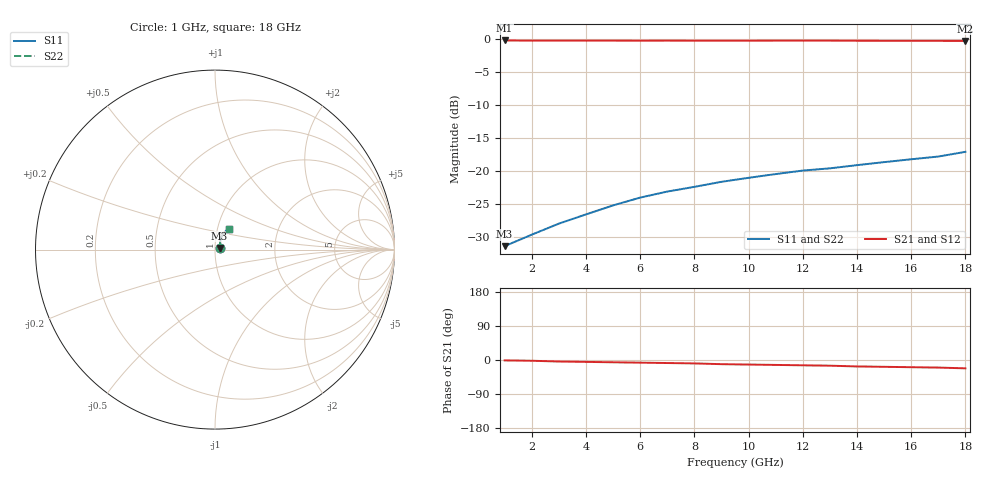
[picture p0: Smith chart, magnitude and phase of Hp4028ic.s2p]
!HPND-4028 beam lead PIN diode
!Series configuration S-parameters If=10 mA.  Last updated 10/3/97
# mhz s ma r 50
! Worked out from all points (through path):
!   18 points, 1 GHz to 18 GHz, reference 50 ohm
!   highest |S21| = -0.19 dB at 1 GHz (marker M1); lowest = -0.3 dB at 18 GHz (marker M2)
!   group delay of S21, straight-line fit = 3.33 ps
!   lowest |S11| = -31.4 dB at 1 GHz (marker M3), VSWR 1.06, Z = 52.6 + j0.926 ohm
!   |S11| at or under -10 dB: start of sweep to end of sweep
!   |S22| runs from -31.4 to -17.1 dB; largest |S21 - S12| = 0
1000  0.027 19.0  0.978 -1.0  0.978 -1.0  0.027 19.0
2000  0.033 37.0  0.975 -2.0  0.975 -2.0  0.033 37.0
3000  0.04 47.0  0.975 -4.0  0.975 -4.0  0.04 47.0
4000  0.047 53.0  0.975 -5.0  0.975 -5.0  0.047 53.0
5000  0.055 58.0  0.975 -6.0  0.975 -6.0  0.055 58.0
6000  0.063 60.0  0.974 -7.0  0.974 -7.0  0.063 60.0
7000  0.07 62.0  0.975 -8.0  0.975 -8.0  0.07 62.0
8000  0.076 63.0  0.974 -9.0  0.974 -9.0  0.076 63.0
9000  0.083 63.0  0.974 -11.0  0.974 -11.0  0.083 63.0
10000  0.089 63.0  0.974 -12.0  0.974 -12.0  0.089 63.0
11000  0.095 63.0  0.975 -13.0  0.975 -13.0  0.095 63.0
12000  0.101 62.0  0.975 -14.0  0.975 -14.0  0.101 62.0
13000  0.105 62.0  0.975 -15.0  0.975 -15.0  0.105 62.0
14000  0.111 61.0  0.973 -17.0  0.973 -17.0  0.111 61.0
15000  0.117 60.0  0.972 -18.0  0.972 -18.0  0.117 60.0
16000  0.123 60.0  0.972 -19.0  0.972 -19.0  0.123 60.0
17000  0.129 57.0  0.971 -20.0  0.971 -20.0  0.129 57.0
18000  0.14 56.0  0.97 -22.0  0.97 -22.0  0.14 56.0
